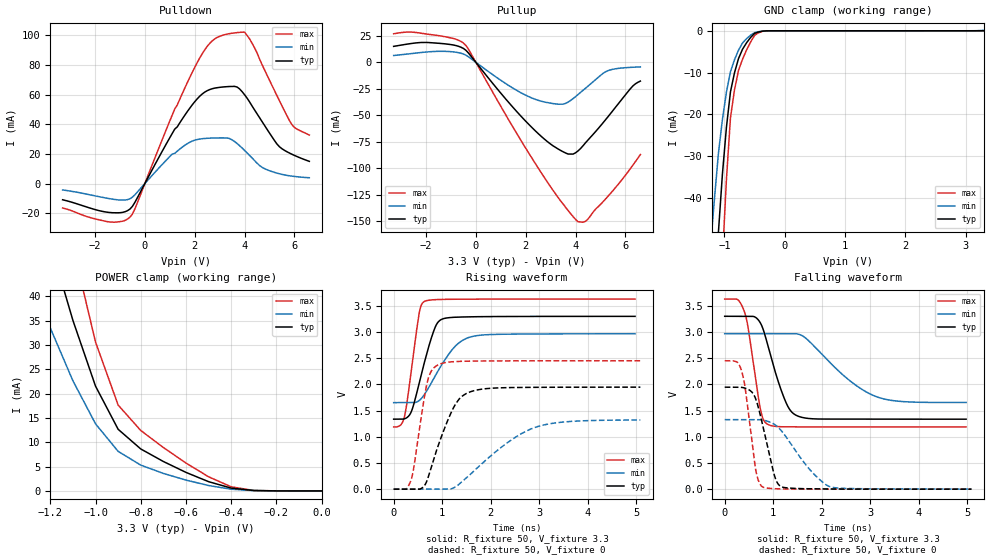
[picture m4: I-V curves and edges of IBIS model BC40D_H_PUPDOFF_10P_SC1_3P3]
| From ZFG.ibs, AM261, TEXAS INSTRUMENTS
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[Model]   BC40D_H_PUPDOFF_10P_SC1_3P3
Model_type   I/O
Polarity   Non-Inverting
Enable   Active-Low
Vinl =  0.8V
Vinh =  2V
Cref =  15pF
Rref =  100.0000M
Vref =  0V
Vmeas =  1.65
C_comp   2.157014p   1.997104p   2.250886p
|[Input load] weak_pupdoff
|[Output drive] slow
|[supplytol] 10
|[temp] ind
[Model Spec]
Vinl   0.8V   0.8V   0.8V
Vinh   2V   2V   2V
[Temperature Range]   25   125   -40
[Voltage Range]   3.3   2.97   3.63
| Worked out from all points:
|   slope of the pulldown table from 0 to 0.495 V, typ, clamps not added: 31.8 ohm
|   slope of the pullup table from 0 to 0.495 V, typ, clamps not added: 33.8 ohm
|   GND clamp passes 1 mA (typ) near -0.53 V on its own axis
|   POWER clamp passes 1 mA (typ) near -0.43 V on its own axis
|   rising waveform, R_fixture 50, V_fixture 3.3: 20-80 % time 338ps typ, 538ps min, 211ps max; typ from 1.34 V to 3.3 V
|   rising waveform, R_fixture 50, V_fixture 0: 20-80 % time 469ps typ, 1.07ns min, 246ps max; typ from 0 V to 1.95 V
|   falling waveform, R_fixture 50, V_fixture 3.3: 20-80 % time 389ps typ, 938ps min, 235ps max; typ from 3.3 V to 1.34 V
|   falling waveform, R_fixture 50, V_fixture 0: 20-80 % time 295ps typ, 648ps min, 202ps max; typ from 1.95 V to 0 V
| Nom Voltages:
|   VDD=1.1001, VDDS=3.3, VDDS18=1.8, ESD_BIASFET=0, VSS=0, VSSS=0
| Min Voltages:
|   VDD=0.99, VDDS=2.97, VDDS18=1.62, ESD_BIASFET=0, VSS=0, VSSS=0
| Max Voltages:
|   VDD=1.21, VDDS=3.63, VDDS18=1.98, ESD_BIASFET=0, VSS=0, VSSS=0
[POWER_clamp]
|   voltage   I(typ)   I(min)   I(max)
-3.3V     446.9mA    419.5mA    603.9mA
-1.267V   62.17mA    41.5mA     88.03mA
-1.233V   56.52mA    37.5mA     80.22mA
-1.133V   40.34mA    26.27mA    57.61mA
-1.067V   30.56mA    19.7mA     43.68mA
-1.033V   26.05mA    16.75mA    37.15mA
-1V       21.55mA    13.8mA     30.62mA
-900mV    12.68mA    8.135mA    17.65mA
-800mV    8.63mA     5.309mA    12.43mA
-600mV    3.813mA    2.231mA    5.733mA
-400mV    580.7uA    357.1uA    842.6uA
0V        4.589uA    2.009uA    9.301uA
[Pulldown]
|   voltage   I(typ)   I(min)   I(max)
-3.3V     -10.93mA   -4.311mA   -16.48mA
-1.4V     -19.53mA   -10.23mA   -25.96mA
-600mV    -17.23mA   -10.26mA   -22.66mA
1.1V      33.82mA    19.89mA    46.25mA
2V        55.14mA    29.24mA    78.29mA
2.6V      63.35mA    30.61mA    94.45mA
3.2V      65.21mA    30.77mA    100.4mA
3.7V      65.09mA    27.02mA    101.8mA
4V        59.92mA    22.37mA    102.1mA
5.3V      26.68mA    7.058mA    59.31mA
5.9V      19.77mA    5.007mA    39.76mA
6.6V      14.97mA    3.923mA    32.7mA
[Pullup]
|   voltage   I(typ)   I(min)   I(max)
-3.3V     15.12mA    6.498mA    27.02mA
-1.9V     18.73mA    9.943mA    26.53mA
-900mV    16.4mA     9.888mA    22.58mA
-400mV    11.39mA    6.786mA    15.98mA
1.3V      -37.44mA   -21.62mA   -53.74mA
2.4V      -65.08mA   -35.06mA   -96.18mA
3.5V      -84.52mA   -39.53mA   -134mA
4.1V      -83.69mA   -30.35mA   -150.6mA
4.4V      -75.99mA   -24.42mA   -150.3mA
5.3V      -51.41mA   -7.872mA   -126.6mA
6.3V      -22.29mA   -4.606mA   -97.15mA
6.6V      -17.71mA   -4.277mA   -87.2mA
[GND_clamp]
|   voltage   I(typ)   I(min)   I(max)
-3.3V     -787.2mA   -607.8mA   -1.235A
-1.233V   -85.66mA   -52.14mA   -138.8mA
-1.167V   -66.47mA   -40.37mA   -107.7mA
-1.1V     -48.25mA   -29.37mA   -77.98mA
-1.033V   -34.27mA   -21.19mA   -54.56mA
-966.7mV  -23.06mA   -14.66mA   -35.51mA
-900mV    -14.61mA   -9.789mA   -20.83mA
-833.3mV  -10.05mA   -6.934mA   -14.15mA
-700mV    -4.416mA   -2.931mA   -6.811mA
-500mV    -621.6uA   -443.4uA   -1.094mA
-300mV    -17.13uA   -24.29uA   -23.57uA
3.3V      4.589uA    110.6uA    5.608uA
[Ramp]
| variable   typ   min   max
dV/dt_f  1.1805379/0.38937314n 0.79480641/0.94605706n   1.467538/0.2356312n
dV/dt_r   1.174185/0.47076118n 0.80302908/1.0837092n  1.4768804/0.24630855n
R_load = 50
[Rising Waveform]
R_fixture = 50
V_fixture = 3.3
V_fixture_min = 2.97
V_fixture_max = 3.63
|   time   V(typ)   V(min)   V(max)
0s        1.337V     1.652V     1.189V
223.5ps   1.343V     1.652V     1.39V
363.3ps   1.479V     1.652V     2.261V
520.8ps   2.003V     1.688V     3.334V
633.7ps   2.421V     1.808V     3.584V
819.3ps   3.004V     2.101V     3.617V
931.6ps   3.206V     2.285V     3.621V
1.274ns   3.283V     2.734V     3.627V
1.574ns   3.291V     2.904V     3.628V
4.974ns   3.3V       2.968V     3.63V
[Rising Waveform]
R_fixture = 50
V_fixture = 0
V_fixture_min = 0
V_fixture_max = 0
|   time   V(typ)   V(min)   V(max)
0s        0V         0V         0V
251.4ps   0V         0V         0V
352.4ps   0V         0V         159.1mV
564.3ps   10.44mV    0V         1.355V
692.5ps   176mV      0V         2.041V
911.4ps   815.3mV    0V         2.371V
1.288ns   1.644V     52.78mV    2.437V
1.63ns    1.874V     326.1mV    2.446V
2.951ns   1.945V     1.19V      2.451V
5.084ns   1.948V     1.321V     2.452V
[Falling Waveform]
R_fixture = 50
V_fixture = 3.3
V_fixture_min = 2.97
V_fixture_max = 3.63
|   time   V(typ)   V(min)   V(max)
0s        3.3V       2.969V     3.629V
266.3ps   3.3V       2.969V     3.619V
404.6ps   3.3V       2.969V     3.392V
481.9ps   3.3V       2.969V     3.087V
738ps     3.169V     2.969V     1.52V
886.5ps   2.752V     2.969V     1.238V
1.253ns   1.675V     2.969V     1.19V
1.517ns   1.391V     2.959V     1.189V
3.08ns    1.337V     1.782V     1.188V
4.974ns   1.336V     1.656V     1.188V
[Falling Waveform]
R_fixture = 50
V_fixture = 0
V_fixture_min = 0
V_fixture_max = 0
|   time   V(typ)   V(min)   V(max)
0s        1.947V     1.328V     2.451V
250.2ps   1.947V     1.328V     2.429V
350.9ps   1.943V     1.328V     2.249V
430.3ps   1.925V     1.328V     1.874V
642.2ps   1.715V     1.328V     351.3mV
785.7ps   1.21V      1.32V      39.33mV
1.034ns   232.5mV    1.232V     8.191mV
1.187ns   39.95mV    1.093V     4.403mV
2.173ns   3.793mV    47.02mV    0V
5.084ns   0V         2.085mV    0V
